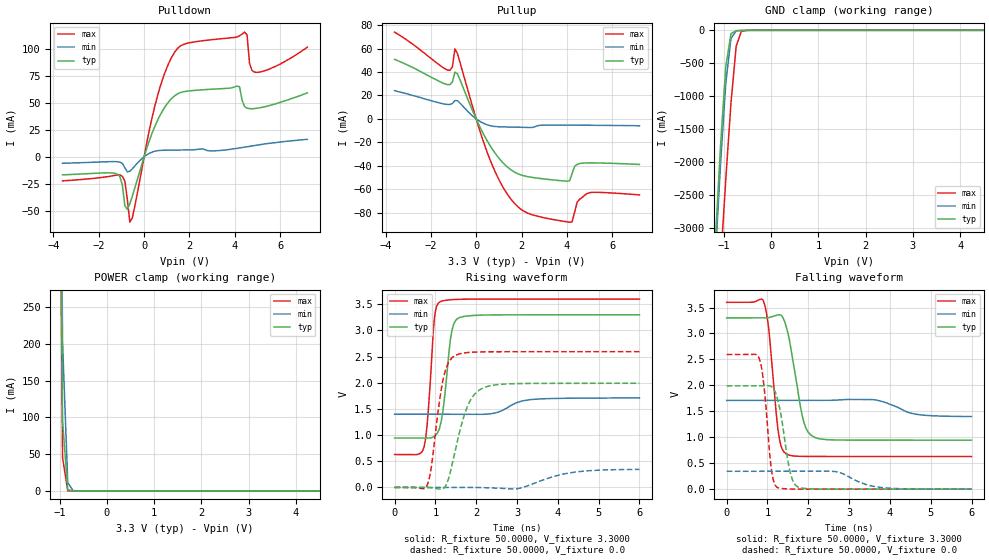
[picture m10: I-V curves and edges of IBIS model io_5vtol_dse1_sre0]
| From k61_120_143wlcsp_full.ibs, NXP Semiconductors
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[Model]  io_5vtol_dse1_sre0
|   Model io_5vtol_dse1_sre0
| Library cells for typ/min/max conditions are connected as defined below:
|  pad - External Pad
|  ipp_do - Core Input
|  ipp_obe - Output Buffer Enable
|  esd_boost - vdd_s_3v
|  esd_bus - vdd_s_3v
|  ipp_ame - vss_s_lv
|  ipp_dse - vdd_s_lv
|  ipp_ina40a_5vtol - NC
|  ipp_ina40b_5vtol - NC
|  ipp_ina_5vtol - NC
|  ipp_ina_mux_3v - NC
|  ipp_ind - NC
|  ipp_ind_3v - NC
|  ipp_pue - vss_s_lv
|  ipp_sre - vss_s_lv
|  tie_3v - vdd_s_3v
|  tie_hi - vdd_s_lv
|  vbuf_3v - vdd_s_3v
|  vdd_bulk_lv - vdd_s_lv
|  vdd_s_3v - vdd_s_3v
|  vdd_s_lv - vdd_s_lv
|  vss_bulk - vss_s_3v
|  vss_s_3v - vss_s_3v
|  vss_s_lv - vss_s_lv
| All other pins connected to ground
Model_type I/O
Polarity   Non-Inverting
Enable   Active-High
Vinl =   1.1550V
Vinh =   2.3100V
Vmeas =  1.6500V
Cref =   25.0000pF
Rref =   50.0000
Vref =   0.0V
C_comp   2.8049pF   2.7887pF   2.9184pF
[Temperature Range]   25.0000   0.1250k   -40.0000
[Voltage Range]   3.3000V   1.7100V   3.6000V
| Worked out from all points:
|   slope of the pulldown table from 0 to 0.495 V, typ, clamps not added: 16.9 ohm
|   slope of the pullup table from 0 to 0.495 V, typ, clamps not added: 26 ohm
|   GND clamp passes 1 mA (typ) near -0.58 V on its own axis
|   POWER clamp passes 1 mA (typ) near -0.79 V on its own axis
|   rising waveform, R_fixture 50.0000, V_fixture 3.3000: 20-80 % time 194ps typ, 495ps min, 150ps max; typ from 0.944 V to 3.3 V
|   rising waveform, R_fixture 50.0000, V_fixture 0.0: 20-80 % time 413ps typ, 888ps min, 270ps max; typ from 0 V to 1.99 V
|   falling waveform, R_fixture 50.0000, V_fixture 3.3000: 20-80 % time 304ps typ, 564ps min, 205ps max; typ from 3.3 V to 0.944 V
|   falling waveform, R_fixture 50.0000, V_fixture 0.0: 20-80 % time 246ps typ, 607ps min, 172ps max; typ from 1.99 V to 0 V
[Pulldown]
|Voltage   I(typ)   I(min)   I(max)
-3.6V     -16.8mA    -6.04mA    -22.41mA
-960mV    -26.33mA   -6.165mA   -18.18mA
-850mV    -45.49mA   -10.24mA   -22.59mA
-630mV    -43.55mA   -13.55mA   -60.83mA
580mV     33.33mA    5.622mA    55.77mA
1.46V     58.28mA    6.234mA    100.4mA
4.1V      65.72mA    7.8mA      111.4mA
4.43V     46.8mA     9mA        115.9mA
4.54V     45.21mA    9.3mA      113.3mA
4.65V     44.72mA    9.6mA      86.87mA
4.98V     45.1mA     10.8mA     78.42mA
7.2V      59.4mA     16.2mA     102mA
[Pullup]
|Voltage   I(typ)   I(min)   I(max)
-3.6V     50.7mA     24.1mA     74mA
-1.27V    29.24mA    12.33mA    41.65mA
-1.05V    31.45mA    13.15mA    44.42mA
-940mV    39.86mA    15.56mA    59.68mA
710mV     -25.74mA   -6.141mA   -39.48mA
1.37V     -40.86mA   -6.889mA   -64.05mA
2.03V     -48.09mA   -7.153mA   -77.75mA
4.12V     -52.71mA   -5.28mA    -88mA
4.34V     -40.52mA   -5.31mA    -79.47mA
4.45V     -38.73mA   -5.32mA    -70.98mA
4.89V     -37.5mA    -5.39mA    -63.55mA
7.2V      -38.79mA   -5.82mA    -64.73mA
[GND_clamp]
|Voltage   I(typ)   I(min)   I(max)
-3.6V     -39.79A    -39.79A    -41.16A
-1.18V    -3.193A    -3.444A    -4.927A
-1.07V    -1.746A    -2.021A    -3.54A
-960mV    -554.7mA   -808.1mA   -2.265A
-850mV    -51.43mA   -125.2mA   -1.104A
-740mV    -5.185mA   -9.147mA   -242.4mA
-630mV    -1.474mA   -1.195mA   -14.98mA
-520mV    -384.8uA   -298.7uA   -1.148mA
7.2V      0A         0A         0A
[POWER_clamp]
|Voltage   I(typ)   I(min)   I(max)
-3.6V     45.62A     45.23A     45.93A
-1.05V    987.4mA    1.121A     927.4mA
-940mV    95.32mA    202.8mA    45.29mA
-830mV    1.645mA    11.46mA    218.1uA
-720mV    22.84uA    474.3uA    919.1nA
-610mV    316.6nA    19.24uA    4.178nA
7.2V      0A         0A         0A
[Ramp]
| variable   typ   min   max
dV/dt_r  1.1940/0.4135n   0.2064/0.8882n   1.5562/0.2701n
dV/dt_f  1.4135/0.3044n   0.1859/0.5641n   1.7827/0.2050n
R_load = 50.0000
[Rising Waveform]
R_fixture= 50.0000
V_fixture= 3.3000
V_fixture_min= 1.7100
V_fixture_max= 3.6000
|time   V(typ)   V(min)   V(max)
0s        943.7mV    1.399V     628.5mV
724.5ps   943.4mV    1.399V     779.7mV
823.1ps   942mV      1.399V     1.434V
976.5ps   979.3mV    1.399V     3.241V
1.103ns   1.136V     1.399V     3.542V
1.223ns   1.706V     1.399V     3.572V
1.37ns    2.836V     1.399V     3.586V
1.544ns   3.227V     1.399V     3.594V
3.364ns   3.299V     1.681V     3.599V
6ns       3.3V       1.71V      3.6V
[Rising Waveform]
R_fixture= 50.0000
V_fixture= 0.0
V_fixture_min= 0.0
V_fixture_max= 0.0
|time   V(typ)   V(min)   V(max)
0s        463.5pV    70.74nV    297.1pV
795.5ps   -747.2uV   1.062uV    39.81mV
908ps     -9.107mV   -3.707uV   430.8mV
1.066ns   -27.33mV   -10.54uV   1.452V
1.198ns   -19.54mV   6.733uV    2.096V
1.309ns   133.1mV    51.51uV    2.368V
1.479ns   680.5mV    184.4uV    2.518V
1.778ns   1.537V     308.8uV    2.577V
2.194ns   1.91V      -4.821mV   2.591V
6ns       1.99V      344mV      2.594V
[Falling Waveform]
R_fixture= 50.0000
V_fixture= 3.3000
V_fixture_min= 1.7100
V_fixture_max= 3.6000
|time   V(typ)   V(min)   V(max)
0s        3.3V       1.71V      3.6V
903.7ps   3.3V       1.71V      3.617V
1.031ns   3.306V     1.71V      3.088V
1.256ns   3.357V     1.71V      1.152V
1.325ns   3.356V     1.71V      847.3mV
1.451ns   3.154V     1.71V      683.1mV
1.848ns   1.429V     1.71V      631.5mV
2.109ns   1.019V     1.71V      630mV
3.585ns   944.8mV    1.726V     629mV
6ns       944.2mV    1.4V       628.9mV
[Falling Waveform]
R_fixture= 50.0000
V_fixture= 0.0
V_fixture_min= 0.0
V_fixture_max= 0.0
|time   V(typ)   V(min)   V(max)
0s        1.991V     344.3mV    2.594V
800.2ps   1.99V      344.3mV    2.512V
915.4ps   1.991V     344.3mV    1.972V
1.109ns   1.97V      344.3mV    305mV
1.234ns   1.769V     344.3mV    35.74mV
1.568ns   285.6mV    344.3mV    3.22mV
1.746ns   41.1mV     344.2mV    1.19mV
2.666ns   682.7uV    338.4mV    423.4uV
3.803ns   379.3uV    30.97mV    314.4uV
6ns       285uV      114.5uV    259.4uV
